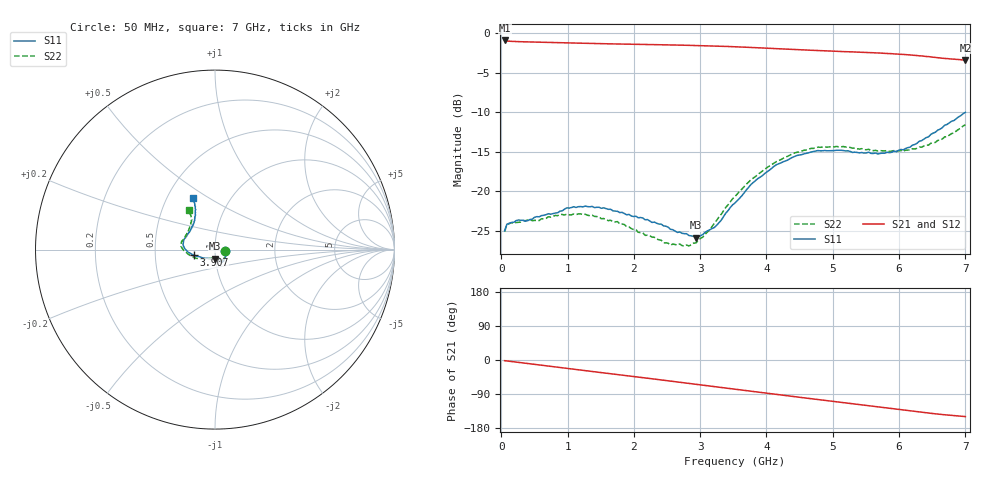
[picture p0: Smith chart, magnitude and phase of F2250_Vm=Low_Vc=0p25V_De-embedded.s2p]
! Integrated Device Technology
! Corporate Headquarters
! 6024 Silver Creek Valley Road
! San Jose, CA 95138  USA
! Phone:  1-408-284-8200
! Toll Free:  1-800-223-1366
! Webpage:  http://www.idt.com/
! Timing and RF Division
! 515 Groton Road, Suite 102
! Westford, MA 01886-6024
! Device:  F2250
! Description: Voltage Variable RF Attenuator
! Frequency:  50.0 -  6000.00 MHz
! Package:  3x3 mm Thin QFN Plastic Package: 16 pin
! Ports:  2 RF, 3 DC
!  Pin  1  = GND
!  Pin  2  = NC
!  Pin  3  = RF1  = Port 1
!  Pin  4  = NC
!  Pin  5  = GND
!  Pin  6  = GND
!  Pin  7  = GND
!  Pin  8  = GND
!  Pin  9  = NC
!  Pin 10  = RF2  = Port 2
!  Pin 11  = NC
!  Pin 12  = GND
!  Pin 13  = GND
!  Pin 14  = VCNTRL
!  Pin 15  = VDD
!  Pin 16  = VMODE
! Vcntrl:  0.250 Volts
! Vmode:  +0.000 Volts
! Vdd:  +3.30  Volts
! Current:  1.108 mA
! Data:  The device was measured on a the F2250 evaluation board which has
!  individual transmission lines to the RF pins.  Data was collected
!  using a calibrated network analyzer.  The evaluation board was
!  de-embedded using a TRL calibration technique.
!  The reference plane is the edge of the package pin.
! Misc:  SN 10
!  Action Tracker AT0258
! Date Measured:  2014-11-26
! Date:  2015-10-15  MJV
! Note:
!  Integrated Device Technology supplies this data as a sample of measured
!  data at the package pin for this product.  Your particular data for this
!  product may vary.
!  Data was taken at 25 degrees C.
!  Integrated Device Technology reserves the right to change this data at anytime.
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# GHz S dB R 50
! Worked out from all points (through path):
!   201 points, 50 MHz to 7 GHz, reference 50 ohm
!   highest |S21| = -0.94 dB at 50 MHz (marker M1); lowest = -3.4 dB at 7 GHz (marker M2)
!   group delay of S21, straight-line fit = 60 ps
!   lowest |S11| = -25.9 dB at 2.934 GHz (marker M3), VSWR 1.11, Z = 49.6 - j5.07 ohm
!   |S11| at or under -10 dB: start of sweep to end of sweep
!   |S22| runs from -26.9 to -11.6 dB; largest |S21 - S12| = 0.00038
!   S11 on the Smith chart (normalised r, x): 50 MHz: 1.12, -0.02; 3.907 GHz: 0.79, -0.05; 7 GHz: 0.67, +0.43
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0.05  -24.97 -9.6  -0.94 -1.8  -0.93 -1.8  -25.09 -10.0
0.08475  -24.16 -9.5  -1.00 -2.5  -1.00 -2.5  -24.22 -9.3
0.15425  -23.93 -11.8  -1.05 -4.0  -1.05 -4.0  -23.98 -11.0
0.57125  -23.23 -29.8  -1.15 -13.1  -1.15 -13.1  -23.70 -30.3
0.884  -22.51 -45.5  -1.22 -19.9  -1.21 -19.9  -22.94 -46.6
1.2315  -21.97 -55.6  -1.29 -27.4  -1.29 -27.4  -22.94 -59.5
1.75275  -22.53 -62.4  -1.38 -38.4  -1.38 -38.4  -23.83 -66.5
2.37825  -24.14 -63.2  -1.47 -51.8  -1.47 -51.8  -26.14 -68.0
2.552  -24.81 -67.3  -1.50 -55.6  -1.50 -55.6  -26.80 -73.6
2.83  -25.59 -82.6  -1.55 -61.7  -1.55 -61.7  -26.91 -92.7
2.93425  -25.85 -91.7  -1.57 -64.0  -1.57 -64.0  -26.53 -101.5
3.21225  -24.58 -121.2  -1.64 -70.2  -1.63 -70.2  -24.07 -127.4
3.525  -21.48 -147.7  -1.73 -77.1  -1.73 -77.1  -20.66 -146.3
3.76825  -19.12 -160.8  -1.82 -82.5  -1.82 -82.5  -18.52 -156.6
3.90725  -18.20 -165.2  -1.88 -85.5  -1.87 -85.5  -17.63 -162.7
4.1505  -16.63 -173.4  -1.97 -90.8  -1.98 -90.8  -16.24 -171.3
4.7065  -14.98 172.4  -2.18 -102.8  -2.19 -102.8  -14.58 175.7
5.15825  -14.84 161.7  -2.34 -112.6  -2.34 -112.6  -14.34 166.5
5.85325  -15.11 138.6  -2.59 -127.5  -2.59 -127.5  -14.96 151.5
6.166  -14.42 127.7  -2.76 -134.3  -2.76 -134.3  -14.78 142.6
6.444  -13.12 119.4  -2.97 -140.1  -2.97 -140.1  -14.16 133.3
7  -10.03 113.1  -3.41 -149.4  -3.42 -149.4  -11.58 123.8
